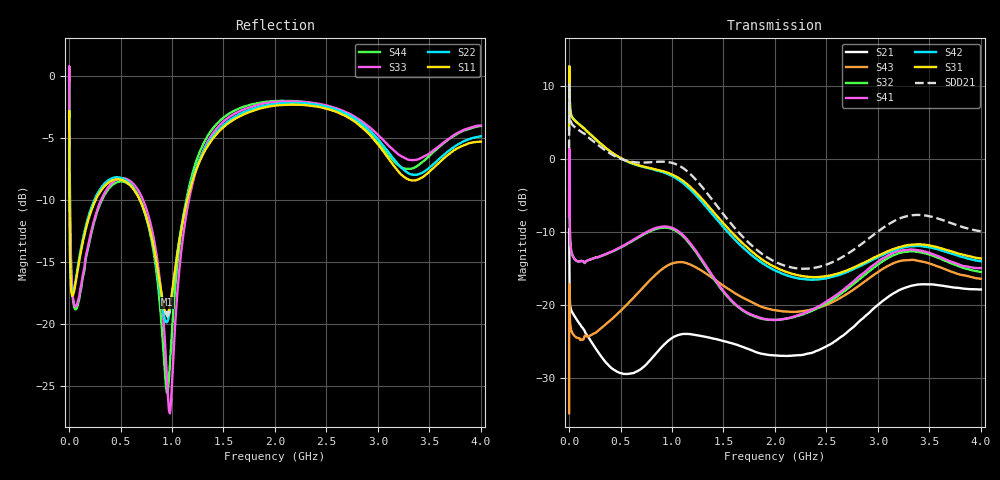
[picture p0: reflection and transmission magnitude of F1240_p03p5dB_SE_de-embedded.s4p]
! Integrated Device Technology
! Corporate Headquarters
! 6024 Silver Creek Valley Road
! San Jose, CA 95138  USA
! Phone:  1-408-284-8200
! Toll Free:  1-800-223-1366
! Webpage:  http://www.idt.com/
! Timing and RF Division
! 515 Groton Road, Suite 102
! Westford, MA 01886-6024
! Device:  F1240
! Description: Dual Intermediate Frequency Digital Variable Gain Amplifier
! Frequency:  10.0 -  500.00 MHz
! Package:  5x5 mm QFN Plastic Package: 32 pin
! Ports:  8 RF, 20 DC
!  Pin  1  = GA3 / Data  Pin 17  = RF OUT_B+
!  Pin  2  = GA4 / CLK  Pin 18  = RF OUT_B-
!  Pin  3  = GA5  Pin 19  = STBY_B
!  Pin  4  = VMODE  Pin 20  = Ground
!  Pin  5  = No Connect  Pin 21  = Ground
!  Pin  6  = GB5  Pin 22  = STB_A
!  Pin  7  = GB4  Pin 23  = RF OUT_A-  = Port 4
!  Pin  8  = GB3  Pin 24  = RF OUT_A+  = Port 3
!  Pin  9  = GB2  Pin 25  = GA0
!  Pin 10  = GB1  Pin 26  = ISET_A
!  Pin 11  = RF IN_B+  Pin 27  = VCC
!  Pin 12  = RF IN_B-  Pin 28  = Ground
!  Pin 13  = Ground  Pin 29  = RF IN_A-  = Port 2
!  Pin 14  = VCC  Pin 30  = RF IN_A+  = Port 1
!  Pin 15  = ISET_B  Pin 31  = GA1
!  Pin 16  = GB0  Pin 32  = GA2 / CSb
! Gain  = +19.5 dB
! State  = 1
! Voltage  = +5.00 V
! Current  = 85.292 mA (one channel only)
! Temperture  =  +25 C
! Test Date  =  2017-10-18
! Board  =  EB4031
! Data:  The device was measured on a custom evaluation board which has
!  individual transmission lines to the RF pins.  Data was collected
!  using a calibrated network analyzer.  The evaluation board was
!  de-embedded using Automatic Fixture Removal.
!  The reference plane is the edge of the package pin.
!  Only Channel A was measured.
!  This data is in single-ended operation.  If your needs are balanced
!  or differential S-parameters then this file needs to be used a
!  linear simulator.
! File Date:  2017-11-10  MJV
! Note:
!  Integrated Device Technology supplies this data as a sample of measured
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# Hz S dB R 100
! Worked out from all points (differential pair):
!   410 points, 500 kHz to 4 GHz, reference 100 ohm
!   strongest paths, dB at 500 kHz, 930 MHz, 1.96 GHz, 2.98 GHz, 4 GHz:
!     S31: 4.1, -1.7, -14.5, -13.3, -13.6
!     S42: 4.1, -1.8, -14.9, -13.5, -14.0
!     S41: -7.8, -9.2, -22.0, -14.3, -14.9
!     S32: -7.8, -9.3, -22.0, -14.6, -15.4
!     S43: -34.8, -14.8, -20.6, -15.6, -16.4
!     S21: -10.0, -25.3, -26.8, -20.2, -17.8
!   taken as a pair (ports 1,2 in; 3,4 out), SDD21 dB: 1.5, -0.3, -13.7, -10.1, -9.8
!   lowest |S11| = -19.2 dB at 950 MHz (marker M1), VSWR 1.25, Z = 81.7 - j7.91 ohm
!   |S11| at or under -10 dB: 4.83 MHz to 257.4 MHz (252.5 MHz wide, 193 % of centre); 688.5 MHz to 1.147 GHz (458.9 MHz wide, 50 % of centre)
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500000  -3.29 -5.5  -9.97 -5.7  -28.88 82.1  -40.68 79.7
        -9.99 -5.7  -3.28 -5.5  -40.67 78.5  -28.87 83.2
        4.09 -105.9  -7.77 -106.6  -0.40 1.2  -34.81 -58.5
        -7.79 -105.5  4.08 -104.8  -34.81 -58.9  -0.41 3.5
2500000  -5.14 -49.3  -13.33 -48.2  -17.95 29.2  -31.67 3.5
         -13.34 -48.2  -5.11 -49.3  -31.63 3.3  -17.95 29.5
         12.27 -178.5  -0.42 158.9  -0.83 -53.9  -17.10 -153.0
         -0.47 159.0  12.27 -178.2  -17.08 -153.1  -0.88 -53.6
4500000  -9.48 -60.8  -17.72 -40.7  -17.86 12.4  -34.15 -10.7
         -17.72 -40.7  -9.43 -61.1  -34.13 -11.1  -17.86 12.5
         9.67 164.0  -6.39 139.0  -4.98 -79.4  -19.57 175.6
         -6.44 139.1  9.67 164.2  -19.54 175.5  -5.04 -79.3
1.8e8  -11.79 -119.6  -24.20 -53.4  -19.92 -46.6  -36.16 -13.2
       -24.21 -53.3  -11.55 -120.9  -36.23 -12.5  -19.93 -46.9
       3.79 113.9  -13.85 61.8  -13.88 -131.0  -24.38 100.9
       -13.84 61.8  3.79 113.2  -24.29 100.3  -14.03 -130.4
5.2e8  -8.39 -168.0  -29.48 -84.8  -21.33 -110.0  -32.01 -67.1
       -29.36 -83.6  -8.25 -169.7  -32.13 -65.0  -21.47 -110.5
       0.06 24.8  -11.94 -56.6  -8.24 -169.1  -20.77 9.5
       -11.88 -57.8  0.01 23.7  -20.50 9.1  -8.50 -169.4
9.5e8  -19.21 -154.1  -25.22 -120.0  -20.25 155.9  -29.27 -155.9
       -25.02 -123.3  -19.86 -152.6  -29.33 -149.9  -20.70 154.6
       -1.79 -82.9  -9.36 171.3  -24.20 168.3  -14.93 -99.3
       -9.21 167.9  -1.95 -85.2  -14.60 -100.0  -25.53 -154.6
4e9  -5.29 -140.7  -17.85 101.9  -24.01 -51.7  -24.88 -34.3
     -17.83 101.6  -4.86 -139.3  -25.72 -18.5  -25.72 -45.5
     -13.58 30.7  -15.41 -75.9  -3.98 -135.5  -17.57 68.7
     -14.90 -89.6  -13.96 36.6  -16.35 58.1  -4.02 -144.8
